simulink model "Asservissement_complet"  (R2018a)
settings: Solver=FixedStepAuto  StartTime=0.0  StopTime=inf  RelTol=1e-3  EnableMultiTasking=on
libraries: arduinolib x4, simulink x2

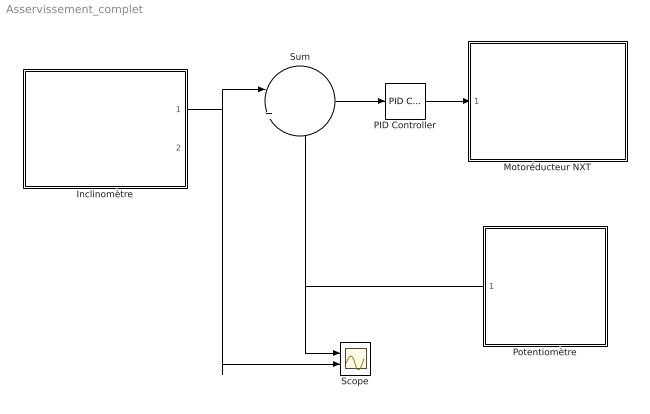
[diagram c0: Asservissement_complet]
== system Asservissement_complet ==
  Inclinomètre : Subsystem
  Motoréducteur NXT : Subsystem
  PID Controller : simulink/Continuous/PID Controller  Controller=PID  TimeDomain=Discrete-time  SampleTime=-1  IntegratorMethod=Forward Euler  FilterMethod=Forward Euler  Form=Parallel  UseFilter=on  ControllerParametersSource=internal  P=0.3  I=0  D=0.025  N=100  InitialConditionSource=internal  InitialConditionForIntegrator=0  InitialConditionForFilter=0  ExternalReset=none  LimitOutput=off  UpperSaturationLimit=inf  LowerSaturationLimit=-inf  LinearizeAsGain=on  AntiWindupMode=none  Kb=1  TrackingMode=off  Kt=1  PParamMin=[]  PParamMax=[]  IParamMin=[]  IParamMax=[]  DParamMin=[]  DParamMax=[]  NParamMin=[]  NParamMax=[]  KbParamMin=[]  KbParamMax=[]  KtParamMin=[]  KtParamMax=[]  POutMin=[]  POutMax=[]  IOutMin=[]  IOutMax=[]  DOutMin=[]  DOutMax=[]  NOutMin=[]  NOutMax=[]  KbOutMin=[]  KbOutMax=[]  KtOutMin=[]  KtOutMax=[]  IntegratorOutMin=[]  IntegratorOutMax=[]  FilterOutMin=[]  FilterOutMax=[]  SumOutMin=[]  SumOutMax=[]  SumI1OutMin=[]  SumI1OutMax=[]  SumI2OutMin=[]  SumI2OutMax=[]  SumI3OutMin=[]  SumI3OutMax=[]  SumDOutMin=[]  SumDOutMax=[]  SaturationOutMin=[]  SaturationOutMax=[]  IntegratorContinuousStateAttributes=''  IntegratorStateMustResolveToSignalObject=off  IntegratorRTWStateStorageClass=Auto  FilterContinuousStateAttributes=''  FilterStateMustResolveToSignalObject=off  FilterRTWStateStorageClass=Auto  DifferentiatorICPrevScaledInput=0  DifferentiatorOutMin=[]  DifferentiatorOutMax=[]  FilterDiffOutCoefMin=[]  FilterDiffOutCoefMax=[]  SumDenOutMin=[]  SumDenOutMax=[]  SumNumOutMin=[]  SumNumOutMax=[]  ReciprocalOutMin=[]  ReciprocalOutMax=[]  DivideOutMin=[]  DivideOutMax=[]  TunerSelectOption=Transfer Function Based (PID Tuner App)
  Potentiomètre : Subsystem
  Scope : Scope  NumInputPorts=2
  Sum : Sum  Inputs=|+-
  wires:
  Potentiomètre/1(Out1) -> Scope/1, Sum/2
  Sum/1 -> PID Controller/1
  PID Controller/1 -> Motoréducteur NXT/1(U)
  Inclinomètre/1(d) -> Scope/2, Sum/1

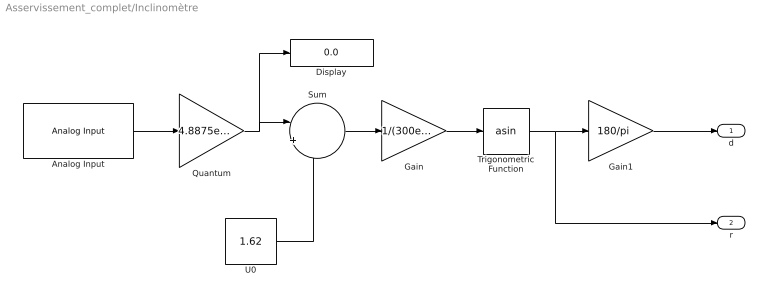
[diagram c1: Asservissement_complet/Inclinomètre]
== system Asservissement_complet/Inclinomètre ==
  Analog Input : arduinolib/Analog Input  pinNumber=4  ReadResultsOnly=off  ConversionTriggerSource=Software  ExternalTriggerType=uint32(0)  OutputDataType=uint16  EnableConversionCompleteNotify=off  EnableOuputStatus=off  SampleTime=0.01  blockPlatform=arduino
  Display : Display
  Gain : Gain  Gain=1/(300e-3)
  Gain1 : Gain  Gain=180/pi
  Quantum : Gain  Gain=4.8875e-3
  Sum : Sum  Inputs=|+-
  Trigonometric Function : Trigonometry  Operator=asin
  U0 : Constant  Value=1.62
  d : Outport
  r : Outport  Port=2
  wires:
  Gain/1 -> Trigonometric Function/1
  Gain1/1 -> d/1
  Trigonometric Function/1 -> r/1, Gain1/1
  Analog Input/1 -> Quantum/1
  U0/1 -> Sum/2
  Quantum/1 -> Display/1, Sum/1
  Sum/1 -> Gain/1

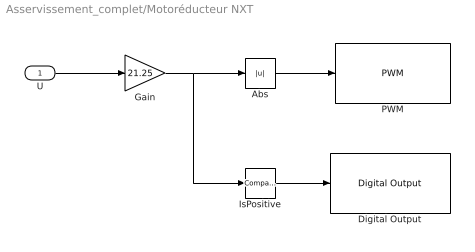
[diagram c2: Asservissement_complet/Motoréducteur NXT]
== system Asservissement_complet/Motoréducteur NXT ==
  U : Inport
  Abs : Abs
  Digital Output : arduinolib/Digital Output  pinNumber=12  blockPlatform=arduino
  Gain : Gain  Gain=21.25
  IsPositive : simulink/Logic and Bit Operations/Compare To Zero  relop=>  OutDataTypeStr=boolean
  PWM : arduinolib/PWM  pinNumber=3  EnableInputFrequency=off  InitialFrequency=2000  InitialDutyCycle=0  NotificationType=None  blockPlatform=arduino
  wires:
  IsPositive/1 -> Digital Output/1
  U/1 -> Gain/1
  Gain/1 -> IsPositive/1, Abs/1
  Abs/1 -> PWM/1

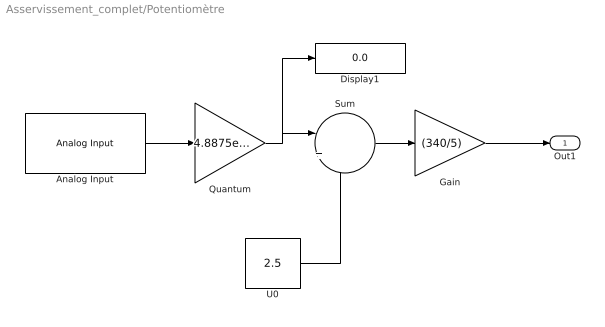
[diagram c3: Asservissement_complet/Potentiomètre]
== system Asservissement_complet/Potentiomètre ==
  Analog Input : arduinolib/Analog Input  pinNumber=5  ReadResultsOnly=off  ConversionTriggerSource=Software  ExternalTriggerType=uint32(0)  OutputDataType=uint16  EnableConversionCompleteNotify=off  EnableOuputStatus=off  SampleTime=0.01  blockPlatform=arduino
  Display1 : Display
  Gain : Gain  Gain=(340/5)
  Quantum : Gain  Gain=4.8875e-3
  Sum : Sum  Inputs=|+-
  U0 : Constant  Value=2.5
  Out1 : Outport
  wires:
  Gain/1 -> Out1/1
  Analog Input/1 -> Quantum/1
  Quantum/1 -> Display1/1, Sum/1
  U0/1 -> Sum/2
  Sum/1 -> Gain/1
